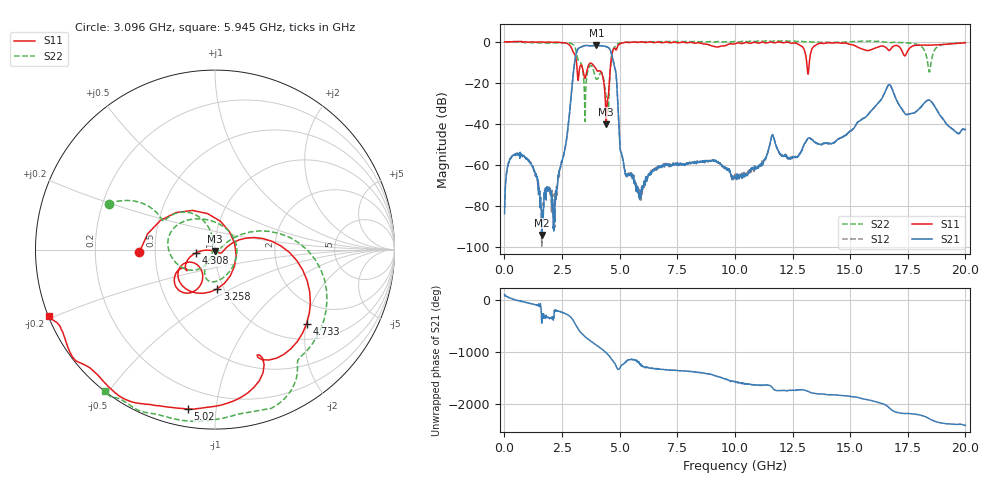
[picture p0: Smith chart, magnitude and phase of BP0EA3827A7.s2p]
! 9/17/2020 12:50:46 PM
! C:\ANRITSUVNA\DATA\MLO\SAMPLES\RAYTHEOM BP\17371_20GH_91720 .S2P
! CHANNEL.1
! TR.MEASUREMENT
! CORRECTED.DATA
# GHZ S RI R 50.0
! FREQ.GHZ  S11RE  S11IM  S31RE  S31IM  S13RE  S13IM  S33RE  S33IM
!; PortSelection: Port_13
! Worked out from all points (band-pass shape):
!   1601 points, 10 MHz to 20 GHz, reference 50 ohm
!   highest |S21| = -1.74 dB at 3.996 GHz (marker M1); lowest = -94.1 dB at 1.622 GHz (marker M2)
!   |S21| within 3 dB of the highest: 3.142 GHz to 4.617 GHz (1.475 GHz wide, 38 % of centre)
!   lowest |S11| = -40.2 dB at 4.42 GHz (marker M3), VSWR 1.02, Z = 50 - j0.98 ohm
!   |S11| at or under -10 dB: 3.129 GHz to 4.619 GHz (1.491 GHz wide, 38.5 % of centre); 13.12 GHz to 13.23 GHz (113.9 MHz wide, 0.864 % of centre)
!   |S22| runs from -38.8 to 0.6 dB; largest |S21 - S12| = 0.0024
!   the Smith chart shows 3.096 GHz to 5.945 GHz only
!   S11 on the Smith chart (normalised r, x): 3.096 GHz: 0.41, -0.01; 3.258 GHz: 0.93, -0.43; 4.308 GHz: 0.81, -0.03; 4.733 GHz: 1.39, -2.01; 5.02 GHz: 0.09, -0.84; 5.945 GHz: 0.00, -0.19
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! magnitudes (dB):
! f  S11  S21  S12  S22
! 10 MHz  0.0  -83.8  -80.9  0.0
! 222.4 MHz  0.0  -57.7  -57.7  0.0
! 634.7 MHz  0.1  -54.2  -54.7  -0.1
! 1.622 GHz  -0.1  -94.1  -99.6  -0.6
! 2.209 GHz  -0.2  -77.0  -79.4  -0.5
! 3.096 GHz  -7.5  -6.9  -6.8  -3.8
! 3.258 GHz  -13.2  -2.9  -2.9  -9.8
! 3.346 GHz  -11.5  -2.5  -2.5  -11.1
! 3.996 GHz  -13.7  -1.7  -1.7  -18.2
! 4.308 GHz  -19.3  -2.0  -2.1  -18.3
! 4.42 GHz  -40.2  -2.4  -2.3  -27.1
! 4.733 GHz  -3.7  -10.0  -10.0  -3.3
! 5.02 GHz  -0.9  -51.8  -51.7  -0.6
! 5.945 GHz  0.0  -71.8  -72.5  0.0
! 6.682 GHz  -0.1  -60.9  -61.4  0.1
! 10.01 GHz  -1.0  -66.8  -64.9  0.2
! 11.63 GHz  -0.3  -45.3  -45.3  0.2
! 13.34 GHz  -3.6  -47.7  -47.5  -0.1
! 16.68 GHz  -4.2  -20.9  -20.9  -0.3
! 17.44 GHz  -5.8  -35.4  -35.5  -0.6
! 18.44 GHz  -1.6  -28.5  -28.4  -14.8
! 20 GHz  -0.5  -42.8  -42.7  -0.3
